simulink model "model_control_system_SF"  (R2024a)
settings: Solver=FixedStepAuto  StartTime=0.0  StopTime=inf  RelTol=1e-3  EnableMultiTasking=on
libraries: lib_control_system_SF x1

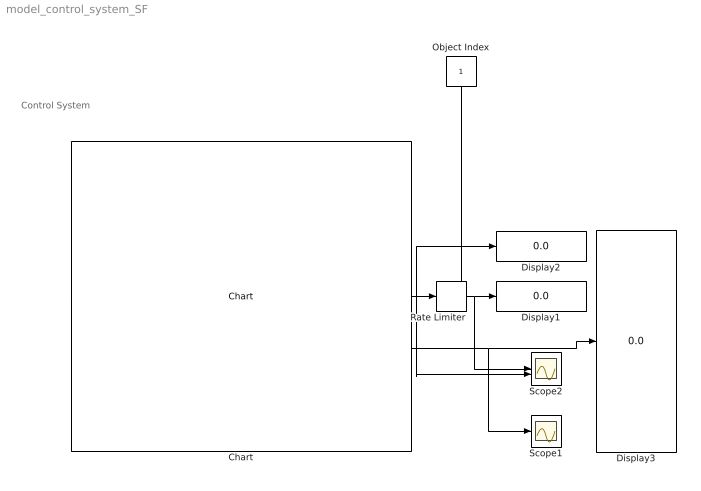
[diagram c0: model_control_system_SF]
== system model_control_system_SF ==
  note: Control System
  Chart : lib_control_system_SF/Chart  SystemSampleTime=-1  VariantActivationTime=update diagram  AllowFlexibleInterface=on  Latency=0  AutoFrameSizeCalculation=off
  Display1 : Display
  Display2 : Display
  Display3 : Display
  Object Index : Constant
  Rate Limiter : RateLimiter  RisingSlewLimit=15  FallingSlewLimit=-15  SampleTimeMode=inherited
  Scope1 : Scope
  Scope2 : Scope  NumInputPorts=2
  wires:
  Chart/1 -> Scope2/2, Display2/1, Rate Limiter/1
  Chart/2 -> Display3/1, Scope1/1
  Rate Limiter/1 -> Scope2/1, Display1/1
  Object Index/1 -> Chart/1
